| Teraspeed Modeling Services.
| http://www.teraspeed.com
[IBIS Ver] 3.0
[File Name] ads5400hfg.ibs
[File Rev] 3.3
[Date]   08-28-2013
|   Modified 05-13-2015 to add ceramic HFG parasitics.  WVB
[Notes]  Quality Check of this IBIS model: Model Passes IBIS Check. Model
   parses into ICX IS. Simulates with Hyperlynx.
   1. MIN TYP MAX information is based on Temperature and Voltage
   characteristics only.
   2. Package information extracted using Tektronix IConnect Software.
   3. Changed topology of CLKINP (N) termination 06-04-2012
   4. For the users of Hyperlynx 9.0,  There was a change in the Hyperlynx
   parser that causes it not to recognize the Model Selector for a series
   termination.  This model has a no_term, 100ohm and 200ohm back term
   associated with the LVDS driver.  For Hyperlynx 9.0 comment out the
   no_term, 100ohm and 200ohm Model statement and enable the out_term
   designation associated with the model you want to use.
   For example to use the 100 Ohm termination:
   |[Model]   no_term
   |[Model]   out_term
   Model_type   Series
   C_comp   0  0  0
   [Voltage Range]  3.3V   3.0V   3.6V
   [Temperature Range] 25   85   -40
   [R series]   10M   10M   10M
[Component] ADS5400
[Manufacturer] TI
[Package]
| variable   typ   min   max
R_pkg  1.837E-02   1.414E-02   2.326E-02
L_pkg  1.102E-09   8.485E-10   1.396E-09
C_pkg  3.062E-13   2.357E-13   3.877E-13
[Pin] signal_name  model_name  R_pin  L_pin C_pin
1   AVDD5   POWER   2.326E-02 1.396E-09 3.877E-13
2   AVDD3   POWER   2.236E-02 1.342E-09 3.727E-13
3   AGND   GND   2.147E-02 1.288E-09 3.579E-13
4   CLKINP   analog   2.059E-02 1.236E-09 3.432E-13
5   CLKINN   analog   1.972E-02 1.183E-09 3.287E-13
6   AGND   GND   1.887E-02 1.132E-09 3.145E-13
7   AVDD3   POWER   1.803E-02 1.082E-09 3.005E-13
8   AGND   GND   1.721E-02 1.032E-09 2.867E-13
9   AVDD5   POWER   1.640E-02 9.841E-10 2.734E-13
10  RESETN   in_lvds   1.562E-02 9.372E-10 2.603E-13
11  RESETP   in_lvds   1.487E-02 8.920E-10 2.478E-13
12  DB11N   lvds_out  1.414E-02 8.485E-10 2.357E-13
13  DB11P   lvds_out  1.414E-02 8.485E-10 2.357E-13
14  DB10N   lvds_out  1.414E-02 8.485E-10 2.357E-13
15  DB10P   lvds_out  1.487E-02 8.920E-10 2.478E-13
16  DB9N   lvds_out  1.562E-02 9.372E-10 2.603E-13
17  DB9P   lvds_out  1.640E-02 9.841E-10 2.734E-13
18  DB8N   lvds_out  1.721E-02 1.032E-09 2.867E-13
19  DB8P   lvds_out  1.803E-02 1.082E-09 3.005E-13
20  DB7N   lvds_out  1.887E-02 1.132E-09 3.145E-13
21  DB7P   lvds_out  1.972E-02 1.183E-09 3.287E-13
22  DB6N   lvds_out  2.059E-02 1.236E-09 3.432E-13
23  DB6P   lvds_out  2.147E-02 1.288E-09 3.579E-13
24  DVDD3   POWER   2.236E-02 1.342E-09 3.727E-13
25  DGND   GND   2.326E-02 1.396E-09 3.877E-13
26  CLKOUTBN  lvds_out  2.326E-02 1.396E-09 3.877E-13
27  CLKOUTBP  lvds_out  2.236E-02 1.342E-09 3.727E-13
28  DB5N   lvds_out  2.147E-02 1.288E-09 3.579E-13
29  DB5P   lvds_out  2.059E-02 1.236E-09 3.432E-13
30  DB4N   lvds_out  1.972E-02 1.183E-09 3.287E-13
31  DB4P   lvds_out  1.887E-02 1.132E-09 3.145E-13
32  DB3N   lvds_out  1.803E-02 1.082E-09 3.005E-13
33  DB3P   lvds_out  1.721E-02 1.032E-09 2.867E-13
34  DB2N   lvds_out  1.640E-02 9.841E-10 2.734E-13
35  DB2P   lvds_out  1.562E-02 9.372E-10 2.603E-13
36  DB1N   lvds_out  1.487E-02 8.920E-10 2.478E-13
37  DB1P   lvds_out  1.414E-02 8.485E-10 2.357E-13
38  DVDD3   POWER   1.414E-02 8.485E-10 2.357E-13
39  DGND   GND   1.414E-02 8.485E-10 2.357E-13
40  DB0N   lvds_out  1.487E-02 8.920E-10 2.478E-13
41  DB0P   lvds_out  1.562E-02 9.372E-10 2.603E-13
42  OVRBN   lvds_out  1.640E-02 9.841E-10 2.734E-13
43  OVRBP   lvds_out  1.721E-02 1.032E-09 2.867E-13
44  OVRAN   lvds_out  1.803E-02 1.082E-09 3.005E-13
45  OVRAP   lvds_out  1.887E-02 1.132E-09 3.145E-13
46  DA0N   lvds_out  1.972E-02 1.183E-09 3.287E-13
47  DA0P   lvds_out  2.059E-02 1.236E-09 3.432E-13
48  DA1N   lvds_out  2.147E-02 1.288E-09 3.579E-13
49  DA1P   lvds_out  2.236E-02 1.342E-09 3.727E-13
50  DVDD3   POWER   2.326E-02 1.396E-09 3.877E-13
51  DGND   GND   2.326E-02 1.396E-09 3.877E-13
52  DA2N   lvds_out  2.236E-02 1.342E-09 3.727E-13
53  DA2P   lvds_out  2.147E-02 1.288E-09 3.579E-13
54  DA3N   lvds_out  2.059E-02 1.236E-09 3.432E-13
55  DA3P   lvds_out  1.972E-02 1.183E-09 3.287E-13
56  DA4N   lvds_out  1.887E-02 1.132E-09 3.145E-13
57  DA4P   lvds_out  1.803E-02 1.082E-09 3.005E-13
58  DA5N   lvds_out  1.721E-02 1.032E-09 2.867E-13
59  DA5P   lvds_out  1.640E-02 9.841E-10 2.734E-13
60  CLKOUTAN  lvds_out  1.562E-02 9.372E-10 2.603E-13
61  CLKOUTAP  lvds_out  1.487E-02 8.920E-10 2.478E-13
62  DA6N   lvds_out  1.414E-02 8.485E-10 2.357E-13
63  DA6P   lvds_out  1.414E-02 8.485E-10 2.357E-13
64  DVDD3   POWER   1.414E-02 8.485E-10 2.357E-13
65  DGND   GND   1.487E-02 8.920E-10 2.478E-13
66  DA7N   lvds_out  1.562E-02 9.372E-10 2.603E-13
67  DA7P   lvds_out  1.640E-02 9.841E-10 2.734E-13
68  DA8N   lvds_out  1.721E-02 1.032E-09 2.867E-13
69  DA8P   lvds_out  1.803E-02 1.082E-09 3.005E-13
70  DA9N   lvds_out  1.887E-02 1.132E-09 3.145E-13
71  DA9P   lvds_out  1.972E-02 1.183E-09 3.287E-13
72  DA10N   lvds_out  2.059E-02 1.236E-09 3.432E-13
73  DA10P   lvds_out  2.147E-02 1.288E-09 3.579E-13
74  DA11N   lvds_out  2.236E-02 1.342E-09 3.727E-13
75  DA11P   lvds_out  2.326E-02 1.396E-09 3.877E-13
76  AVDD5   POWER   2.326E-02 1.396E-09 3.877E-13
77  SDENB   in_pu   2.236E-02 1.342E-09 3.727E-13
78  SCLK   in_sclk   2.147E-02 1.288E-09 3.579E-13
79  SDIO   spi_io   2.059E-02 1.236E-09 3.432E-13
80  SDO   spi_tri   1.972E-02 1.183E-09 3.287E-13
81  ENA1BUS   in_pd_40k 1.887E-02 1.132E-09 3.145E-13
82  ENPWD   in_pd_50k 1.803E-02 1.082E-09 3.005E-13
83  ENEXTREF  in_pd_50k 1.721E-02 1.032E-09 2.867E-13
84  AGND   GND   1.640E-02 9.841E-10 2.734E-13
85  AVDD3   POWER   1.562E-02 9.372E-10 2.603E-13
86  AVDD5   POWER   1.487E-02 8.920E-10 2.478E-13
87  VREF   POWER   1.414E-02 8.485E-10 2.357E-13
88  AGND   GND   1.414E-02 8.485E-10 2.357E-13
89  VCM   analog1   1.414E-02 8.485E-10 2.357E-13
90  AVDD5   POWER   1.487E-02 8.920E-10 2.478E-13
91  AGND   GND   1.562E-02 9.372E-10 2.603E-13
92  AVDD5   POWER   1.640E-02 9.841E-10 2.734E-13
93  AGND   GND   1.721E-02 1.032E-09 2.867E-13
94  AINP   analog2   1.803E-02 1.082E-09 3.005E-13
95  AINN   analog2   1.887E-02 1.132E-09 3.145E-13
96  AGND   GND   1.972E-02 1.183E-09 3.287E-13
97  AVDD5   POWER   2.059E-02 1.236E-09 3.432E-13
98  AGND   GND   2.147E-02 1.288E-09 3.579E-13
99  AVDD5   POWER   2.236E-02 1.342E-09 3.727E-13
100 AGND   GND   2.326E-02 1.396E-09 3.877E-13
[Diff Pin] inv_pin vdiff tdelay_typ tdelay_min tdelay_max
4   5   600mV  NA   NA   NA
94   95   NA   NA   NA   NA
11   10   350mV  NA   NA   NA
13   12   NA   NA   NA   NA
15   14   NA   NA   NA   NA
17   16   NA   NA   NA   NA
19   18   NA   NA   NA   NA
21   20   NA   NA   NA   NA
23   22   NA   NA   NA   NA
27   26   NA   NA   NA   NA
29   28   NA   NA   NA   NA
31   30   NA   NA   NA   NA
33   32   NA   NA   NA   NA
35   34   NA   NA   NA   NA
37   36   NA   NA   NA   NA
41   40   NA   NA   NA   NA
43   42   NA   NA   NA   NA
45   44   NA   NA   NA   NA
47   46   NA   NA   NA   NA
49   48   NA   NA   NA   NA
53   52   NA   NA   NA   NA
55   54   NA   NA   NA   NA
57   56   NA   NA   NA   NA
59   58   NA   NA   NA   NA
61   60   NA   NA   NA   NA
63   62   NA   NA   NA   NA
67   66   NA   NA   NA   NA
69   68   NA   NA   NA   NA
71   70   NA   NA   NA   NA
73   72   NA   NA   NA   NA
75   74   NA   NA   NA   NA
[Series Pin Mapping] pin_2 model_name function_table_group
4   5   200ohm
11   10   100ohm
13   12   out_term
15   14   out_term
17   16   out_term
19   18   out_term
21   20   out_term
23   22   out_term
27   26   out_term
29   28   out_term
31   30   out_term
33   32   out_term
35   34   out_term
37   36   out_term
41   40   out_term
43   42   out_term
45   44   out_term
47   46   out_term
49   48   out_term
53   52   out_term
55   54   out_term
57   56   out_term
59   58   out_term
61   60   out_term
63   62   out_term
67   66   out_term
69   68   out_term
71   70   out_term
73   72   out_term
75   74   out_term
[Model Selector] lvds_out
lvds_5.5ma  5.5ma lvds output
lvds_4.5ma  4.5ma lvds output
lvds_3.5ma  3.5ma lvds output
lvds_2.5ma  2.5ma lvds output
[Model Selector] out_term
no_term   no internal termination
100ohm   100ohm internal termination
200ohm   200ohm internal termination
   |[Model]   100ohm
   [Model]   out_term
   Model_type   Series
   C_comp   0  0  0
   [Voltage Range]  5.00V   4.75V   5.25V
   [Temperature Range] 25   85   -40
   [R series]   100   90   110
   |[Model]   200ohm
   |[Model]   out_term
   Model_type   Series
   C_comp   0  0  0
   [Voltage Range]  3.3V   3.0V   3.6V
   [Temperature Range] 25   85   -40
   [R series]   200   180   220
[Disclaimer]
| Use: Teraspeed Consulting Group LLC ("Teraspeed") has
| licensed IBIS models to specific integrated circuit
| suppliers ("IC Vendors") for use and distribustion as
| follows: Each IC Vendor may use IBIS Models, and distribute
| them to IC Vendor's custumers to use solely for developing
| printed circute board designs. Users of this model may
| modify the IBIS model to suit its specific applications but
| rights to derivative works and such modifications shell belong
| to Teraspeed. No other distribusion of these materials is
| permitted.
| DISCLAIMER OF WARRANTY: UNLESS OTHERWISE AGREED TO IN WRITING
| TERASPEED DISCLAIMS AND USER WAIVES ALL WARRANTIES, EXPRESS
| OR IMPLIED, INCLUDING WARRANTIES OF MERCHANTABILITY AND
| FITNESS FOR A PARTICULAR PURPOSE. IN NO EVENT SHALL
| TERASPEED BE LIABLE FOR ANY DIRECT OR INDIRECT DAMAGES,
| WHETHER IN CONTRACT OR TORT, INCLUDING, WITHOUT LIMITATION,
| LOST PROFITS, BUSINESS INTERRUPTION, OR LOST INFORMATION
| ARISING OUT OF THE USE OF OR THE INABILITY TO USE THE MODEL,
| EVEN IF TERASPEED HAS BEEN ADVISED OF THE POSSIBILITY OF SUCH
| DAMAGES.
[Source]
| This model file was created by Teraspeed Consulting Group LLC
| (http://www.teraspeed.com/).
[Disclaimer]
| This product is designed as an aid for customers of Texas Instruments.
| No warranties, either expressed or implied, with respect to this third
| party software (if any) or with respect to its fitness for any
| particular purpose is claimed by Texas Instruments or the author. The
| software (if any) is provided solely on an "as is" basis. The entire
| risk as to its quality and performance is with the customer
[Copyright]
| (C) Copyright 2009 Texas Instruments Incorporated. All rights reserved.
| All other rights are reserved.
[Model]  analog
Model_type Terminator
C_comp   0   0   0
[Voltage Range]  2.5  2.375  2.625
[Temperature Range] 25   85   -40
[Rpower]  400  360  440
[Model]  analog1
Model_type Terminator
C_comp   0   0   0
[Voltage Range]  2.5  2.375  2.625
[Temperature Range] 25   85   -40
[Rpower]  50  NA  NA
[Model]  analog2
Model_type Terminator
C_comp   0   0   0
[Voltage Range]  2.5  2.375  2.625
[Temperature Range] 25   85   -40
[Rpower]  50  42.5  57.5
[Model]   no_term
|[Model]   out_term
Model_type   Series
C_comp   0  0  0
[Voltage Range]  3.3V   3.0V   3.6V
[Temperature Range] 25   85   -40
[R series]   10M   10M   10M
[Model]   100ohm
|[Model]   out_term
Model_type   Series
C_comp   0  0  0
[Voltage Range]  5.00V   4.75V   5.25V
[Temperature Range] 25   85   -40
[R series]   100   90   110
[Model]   200ohm
|[Model]   out_term
Model_type   Series
C_comp   0  0  0
[Voltage Range]  3.3V   3.0V   3.6V
[Temperature Range] 25   85   -40
[R series]   200   180   220
| Models and submodels in the file (18): out_term (Series), analog (Terminator), analog1 (Terminator), analog2 (Terminator), no_term (Series), 100ohm (Series), 200ohm (Series), in_lvds (Input), in_pd_40k (Input), in_pd_50k (Input), in_pu (Input), in_sclk (Input), lvds_2.5ma (3-state), lvds_3.5ma (3-state), lvds_4.5ma (3-state), lvds_5.5ma (3-state), spi_io (I/O), spi_tri (3-state)
